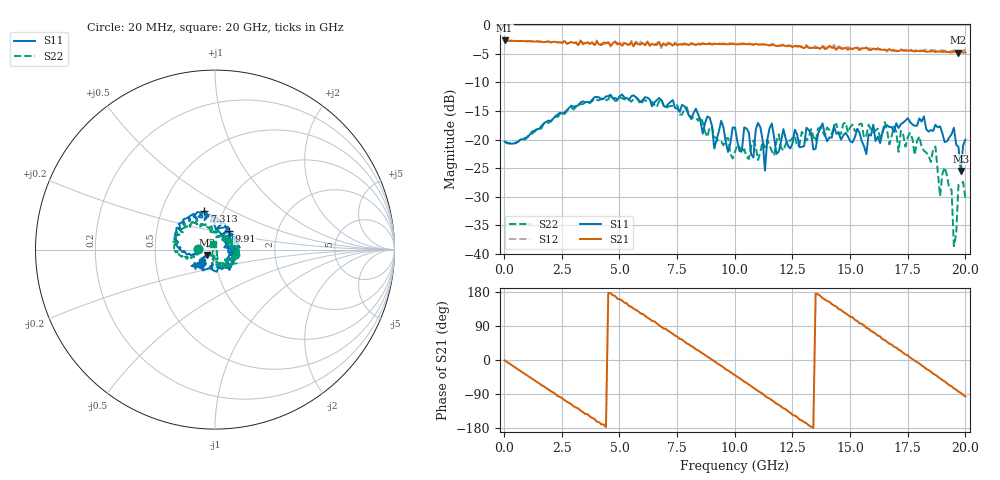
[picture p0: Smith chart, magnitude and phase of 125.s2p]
!Agilent Technologies,N5230A,US43500223,A.07.50.48
!Agilent N5230A: A.07.50.48
!Date: Sunday, September 13, 2015 22:00:45
!Correction: S11(Full 2 Port(1,2))
!S21(Full 2 Port(1,2))
!S12(Full 2 Port(1,2))
!S22(Full 2 Port(1,2))
!S2P File: Measurements: S11, S21, S12, S22:
# Hz S  dB  R 50
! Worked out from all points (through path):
!   201 points, 20 MHz to 20 GHz, reference 50 ohm
!   highest |S21| = -2.65 dB at 20 MHz (marker M1); lowest = -4.8 dB at 19.7 GHz (marker M2)
!   group delay of S21, straight-line fit = 113 ps
!   lowest |S11| = -25.5 dB at 19.8 GHz (marker M3), VSWR 1.11, Z = 45.7 - j2.71 ohm
!   |S11| at or under -10 dB: start of sweep to end of sweep
!   |S22| runs from -38.7 to -12.3 dB; largest |S21 - S12| = 0.05
!   S11 on the Smith chart (normalised r, x): 20 MHz: 0.82, +0.00; 7.313 GHz: 0.81, +0.37; 9.91 GHz: 1.14, +0.24; 20 GHz: 0.85, -0.11
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2e7  -20.36 179.1  -2.65 -0.9  -2.65 -0.9  -20.26 179.1
1.9181e9  -16.67 -171.0  -2.81 -78.0  -2.85 -78.1  -17.09 -161.0
3.4166e9  -13.32 173.2  -3.17 -137.6  -3.39 -139.4  -13.79 -171.7
4.8152e9  -12.73 148.2  -2.82 168.8  -3.01 170.4  -13.23 170.6
6.7133e9  -12.73 114.8  -2.97 92.1  -2.89 91.4  -13.36 142.2
7.3127e9  -13.08 105.5  -3.55 68.9  -3.56 70.5  -14.12 129.8
9.9101e9  -17.90 53.5  -3.25 -36.2  -3.20 -37.4  -23.31 84.0
1.001e10  -17.88 37.2  -3.31 -40.4  -3.19 -41.2  -22.10 76.7
1.08092e10  -23.16 35.7  -3.44 -73.3  -3.34 -74.5  -20.17 48.9
1.1009e10  -17.09 26.7  -3.35 -81.7  -3.37 -83.6  -23.58 56.1
1.13087e10  -25.45 14.7  -3.39 -94.7  -3.38 -96.1  -21.36 36.9
1.16084e10  -17.19 5.2  -3.38 -106.1  -3.25 -107.7  -22.03 19.5
1.34066e10  -21.75 -43.7  -3.90 -179.0  -3.75 -178.8  -19.50 -3.5
1.5005e10  -20.31 -82.9  -4.01 114.2  -3.90 112.1  -17.83 -8.6
1.67033e10  -17.80 -139.4  -4.17 43.2  -4.12 43.0  -20.85 -40.7
1.87013e10  -17.41 -133.4  -4.69 -39.4  -4.41 -42.2  -21.22 -84.7
1.89011e10  -17.69 -138.1  -4.60 -48.2  -4.44 -51.9  -29.92 -91.7
1.94006e10  -19.07 -134.8  -4.78 -69.3  -4.52 -73.3  -28.78 -115.2
1.95005e10  -17.94 -133.2  -4.59 -74.9  -4.39 -77.3  -38.66 -170.3
1.97003e10  -21.29 -146.2  -4.78 -83.3  -4.45 -87.5  -27.93 -74.3
1.98002e10  -25.51 -146.1  -4.69 -87.1  -4.70 -90.1  -27.70 -125.6
2e10  -20.02 -138.1  -4.75 -96.3  -4.31 -100.2  -30.27 106.8
